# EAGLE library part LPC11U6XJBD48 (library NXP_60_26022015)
32-bit ARM Cortex-M0+ microcontroller; up to 256 kB flash and 36 kB SRAM; 4 kB EEPROM; USB; 12-bit ADC The LPC11U6x are an ARM Cortex-M0+ based, low-cost 32-bit MCU family operating at CPU frequencies of up to 50 MHz. The LPC11U6x support up to 256 kB of flash memory, a 4 kB EEPROM, and 36 kB of SRAM. The ARM Cortex-M0+ is an easy-to-use, energy-efficient core using a two-stage pipeline and fast single-cycle I/O access. The peripheral complement of the LPC11U6x includes a DMA controller, a CRC engine, one full-speed USB device controller with XTAL-less low-speed mode, two I2C-bus interfaces, up to five USARTs, two SSP interfaces, PWM/timer subsystem with six configurable multi-purpose timers, a Real-Time Clock, one 12-bit ADC, temperature sensor, function-configurable I/O ports, and up to 80 general-purpose I/O pins. AAL Eindhoven MK
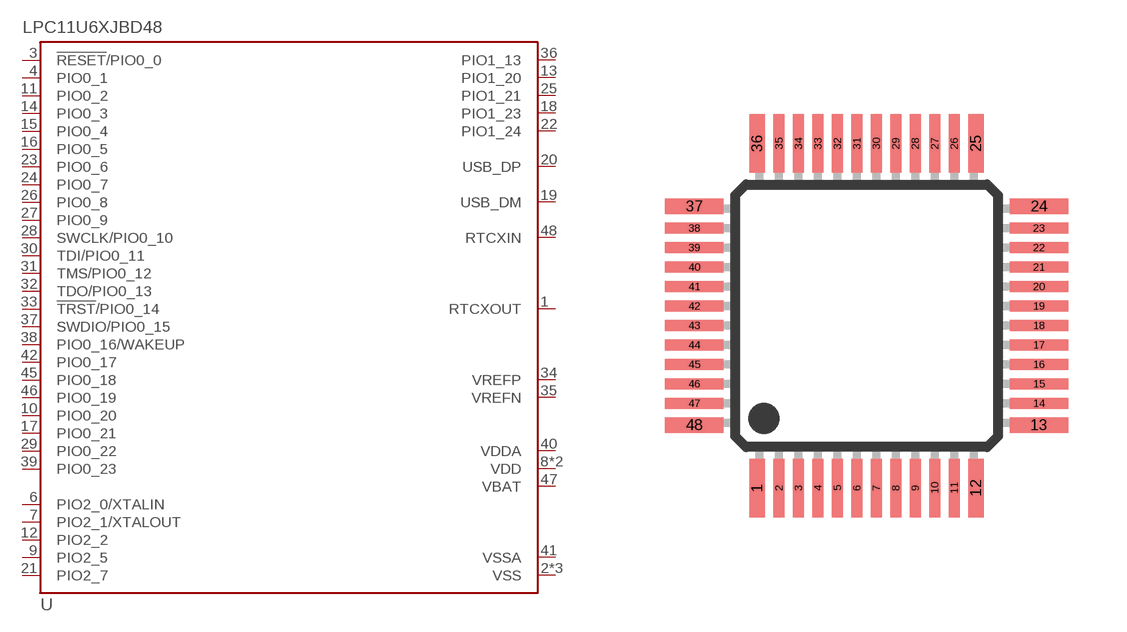
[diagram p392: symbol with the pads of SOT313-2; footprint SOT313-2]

Designator prefix U

## LPC11U6XJBD48  [SOT313-2]
1  RTCXOUT
2  VSS
3  !RESET!/PIO0_0
4  PIO0_1
5  VSS
6  PIO2_0/XTALIN
7  PIO2_1/XTALOUT
8  VDD
9  PIO2_5
10  PIO0_20
11  PIO0_2
12  PIO2_2
13  PIO1_20
14  PIO0_3
15  PIO0_4
16  PIO0_5
17  PIO0_21
18  PIO1_23
19  USB_DM
20  USB_DP
21  PIO2_7
22  PIO1_24
23  PIO0_6
24  PIO0_7
25  PIO1_21
26  PIO0_8
27  PIO0_9
28  SWCLK/PIO0_10
29  PIO0_22
30  TDI/PIO0_11
31  TMS/PIO0_12
32  TDO/PIO0_13
33  !TRST!/PIO0_14
34  VREFP
35  VREFN
36  PIO1_13
37  SWDIO/PIO0_15
38  PIO0_16/WAKEUP
39  PIO0_23
40  VDDA
41  VSSA
42  PIO0_17
43  VSS
44  VDD
45  PIO0_18
46  PIO0_19
47  VBAT
48  RTCXIN

## Footprint SOT313-2 (pad centres in mm)
SOT313-2 LQFP48: plastic low profile quad flat package; 48 leads; body 7 x 7 x 1.4 mm JEDEC: MS-026 IEC: 136E05 Footprint according to NXP SOT313-2 specification, however the cornerpins are 0.4mm in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
smd 0.4 x 1.5: 1 -2.81,-4.425; 12 2.81,-4.425; 25 2.81,4.425; 36 -2.81,4.425
smd 0.28 x 1.5: 2 -2.25,-4.425; 3 -1.75,-4.425; 4 -1.25,-4.425; 5 -0.75,-4.425; 6 -0.25,-4.425; 7 0.25,-4.425; 8 0.75,-4.425; 9 1.25,-4.425; 10 1.75,-4.425; 11 2.25,-4.425; 26 2.25,4.425; 27 1.75,4.425; 28 1.25,4.425; 29 0.75,4.425; 30 0.25,4.425; 31 -0.25,4.425; 32 -0.75,4.425; 33 -1.25,4.425; 34 -1.75,4.425; 35 -2.25,4.425
smd 1.5 x 0.4: 13 4.425,-2.81; 24 4.425,2.81; 37 -4.425,2.81; 48 -4.425,-2.81
smd 1.5 x 0.28: 14 4.425,-2.25; 15 4.425,-1.75; 16 4.425,-1.25; 17 4.425,-0.75; 18 4.425,-0.25; 19 4.425,0.25; 20 4.425,0.75; 21 4.425,1.25; 22 4.425,1.75; 23 4.425,2.25; 38 -4.425,2.25; 39 -4.425,1.75; 40 -4.425,1.25; 41 -4.425,0.75; 42 -4.425,0.25; 43 -4.425,-0.25; 44 -4.425,-0.75; 45 -4.425,-1.25; 46 -4.425,-1.75; 47 -4.425,-2.25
